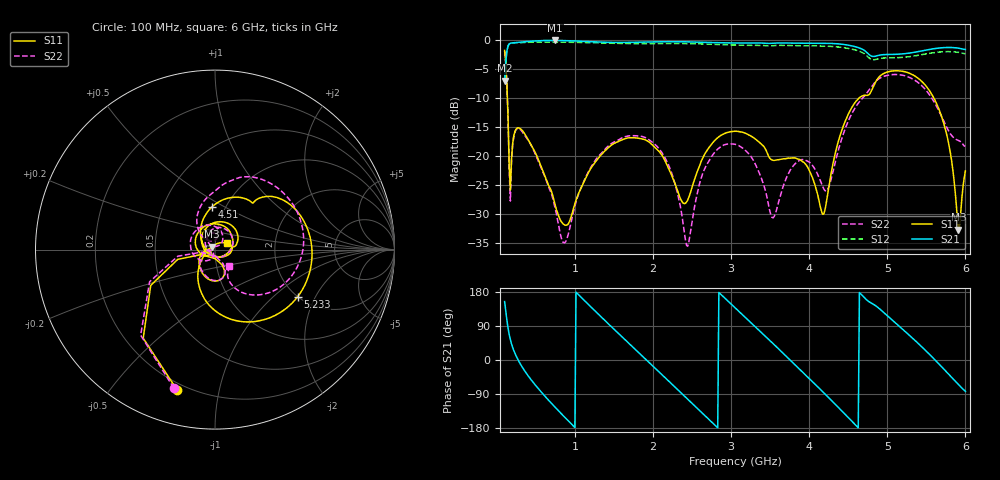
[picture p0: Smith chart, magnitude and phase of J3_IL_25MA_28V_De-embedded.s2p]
!Keysight Technologies,N5242B,MY61256241,Z.15.82.127
!Date: Friday, August 25, 2023 02:23:25
!Correction: S11(C  4-Port  )
!S41(C  4-Port  )
!S14(C  4-Port  )
!S44(C  4-Port  )
!S2P File: Measurements: S11, S41, S14, S44:
# Hz S  dB  R 50
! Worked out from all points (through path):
!   401 points, 100 MHz to 6 GHz, reference 50 ohm
!   highest |S21| = -0.09 dB at 749 MHz (marker M1); lowest = -7.0 dB at 100 MHz (marker M2)
!   group delay of S21, straight-line fit = 555 ps
!   lowest |S11| = -32.7 dB at 5.912 GHz (marker M3), VSWR 1.05, Z = 48.3 + j1.55 ohm
!   |S11| at or under -10 dB: 135.4 MHz to 4.639 GHz (4.504 GHz wide, 189 % of centre); 5.596 GHz to end of sweep
!   |S22| runs from -35.5 to -1.9 dB; largest |S21 - S12| = 0.068
!   S11 on the Smith chart (normalised r, x): 100 MHz: 0.16, -0.75; 4.51 GHz: 0.86, +0.43; 5.233 GHz: 2.00, -1.46; 6 GHz: 1.14, +0.08
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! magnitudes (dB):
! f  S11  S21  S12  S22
! 100 MHz  -1.8  -7.0  -7.1  -1.9
! 159 MHz  -21.8  -0.7  -0.7  -22.5
! 188.5 MHz  -20.5  -0.5  -0.5  -20.9
! 306.5 MHz  -15.3  -0.4  -0.5  -15.5
! 749 MHz  -28.4  -0.1  -0.4  -29.1
! 867 MHz  -31.8  -0.1  -0.4  -34.9
! 1.088 GHz  -25.2  -0.2  -0.4  -25.2
! 1.605 GHz  -17.2  -0.4  -0.6  -16.8
! 2.076 GHz  -19.2  -0.3  -0.6  -18.7
! 2.445 GHz  -27.6  -0.3  -0.6  -35.5
! 2.667 GHz  -19.5  -0.4  -0.7  -22.0
! 3.05 GHz  -15.7  -0.5  -0.9  -18.0
! 3.537 GHz  -20.7  -0.5  -1.0  -30.6
! 3.788 GHz  -20.3  -0.6  -1.0  -21.8
! 4.038 GHz  -23.6  -0.6  -1.0  -21.5
! 4.186 GHz  -30.0  -0.6  -1.1  -25.6
! 4.51 GHz  -12.5  -0.9  -1.5  -13.7
! 5.027 GHz  -5.4  -2.5  -3.1  -6.0
! 5.233 GHz  -5.5  -2.4  -3.0  -6.2
! 5.676 GHz  -12.4  -1.4  -2.1  -12.6
! 5.912 GHz  -32.7  -1.4  -2.1  -17.3
! 6 GHz  -22.6  -1.6  -2.4  -18.3
